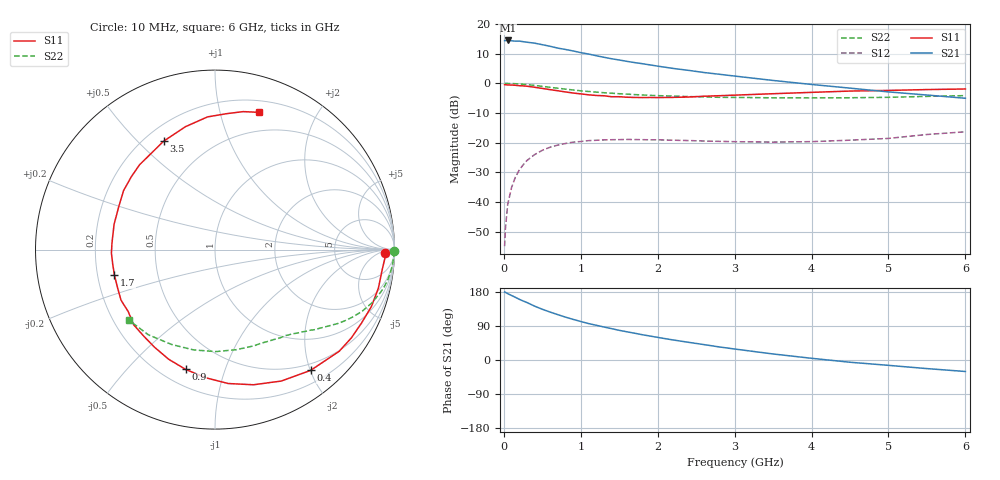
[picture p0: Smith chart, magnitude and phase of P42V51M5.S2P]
! SIEMENS Small Signal Semiconductors
! BFP182
! Si NPN RF Bipolar Junction Transistor in SOT143
! VCE = 2.5 V  IC = 1.5 mA
! Common Emitter S-Parameters:  March  1996
# GHz  S  MA  R  50
!  f  S11  S21  S12  S22
! GHz  MAG  ANG  MAG  ANG  MAG  ANG  MAG  ANG
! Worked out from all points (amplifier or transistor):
!   36 points, 10 MHz to 6 GHz, reference 50 ohm
!   highest |S21| = 14.5 dB at 50 MHz (marker M1)
!   |S21| within 3 dB of that: start of sweep to 793.3 MHz
!   unconditionally stable (mu >= 1): 2.371 GHz to end of sweep
!   at 250 MHz: K = 0.11, MSG = 20.8 dB, |S12| = -27.5 dB
!   at 1.4 GHz: K = 0.61, MSG = 13.6 dB, |S12| = -19.0 dB
!   at 6 GHz: K = 1.02, MAG = 4.8 dB, |S12| = -16.3 dB
!   S11 on the Smith chart (normalised r, x): 10 MHz: 31, -13; 400 MHz: 0.39, -2.01; 900 MHz: 0.29, -0.74; 1.7 GHz: 0.27, -0.12; 3.5 GHz: 0.27, +0.60; 6 GHz: 0.31, +1.33
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0.01  0.9462 -1.3  5.243 179.3  0.0018 94.1  0.9972 -0.5
0.02  0.9487 -2.6  5.242 178.7  0.0035 81.9  0.9974 -1.0
0.05  0.9383 -6.8  5.28 175.1  0.0091 88.4  0.9964 -2.5
0.1  0.9353 -13.3  5.209 170.3  0.0175 80.6  0.992 -5.1
0.2  0.913 -26.7  5.152 160.3  0.0345 74.3  0.9766 -10.1
0.3  0.8944 -39.3  4.935 151.7  0.05 66.6  0.9519 -14.6
0.4  0.8584 -51.6  4.753 142.1  0.0629 60.0  0.9229 -18.8
0.5  0.8203 -63.2  4.479 133.9  0.0743 53.2  0.8899 -22.6
0.6  0.783 -74.1  4.215 126.6  0.0837 47.6  0.8572 -25.8
0.7  0.7497 -84.4  3.924 119.8  0.0909 42.7  0.8277 -28.5
0.8  0.7157 -94.2  3.725 113.2  0.0968 38.1  0.7991 -31.0
0.9  0.6872 -103.8  3.514 107.2  0.102 34.0  0.7722 -33.1
1.1  0.6402 -121.6  3.12 96.2  0.1082 27.3  0.7288 -37.0
1.4  0.5942 -144.4  2.597 82.8  0.1121 19.1  0.6816 -41.9
1.7  0.5782 -165.7  2.237 70.7  0.1128 14.1  0.646 -46.3
1.9  0.5774 -178.1  2.045 63.2  0.1118 11.5  0.628 -49.2
2.2  0.5796 165.9  1.784 52.9  0.11 8.4  0.6108 -53.7
2.8  0.6183 138.9  1.422 34.5  0.1052 6.4  0.5812 -63.8
3.5  0.6684 115.4  1.118 15.9  0.1022 7.6  0.5702 -78.0
4.5  0.7406 93.2  0.83 -5.9  0.1101 13.3  0.5715 -102.1
5.5  0.7848 78.4  0.635 -22.7  0.1373 16.8  0.6026 -128.0
6  0.8032 72.2  0.56 -30.3  0.1524 14.6  0.6207 -140.8
